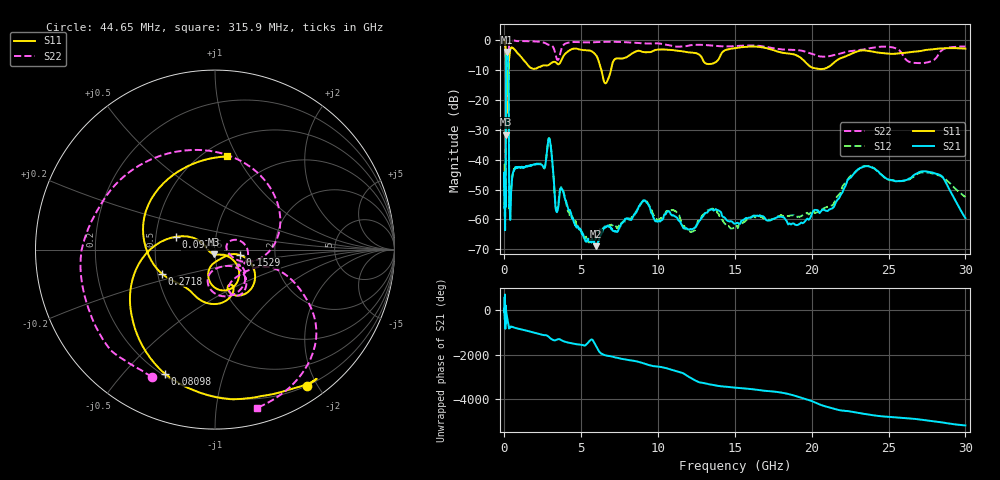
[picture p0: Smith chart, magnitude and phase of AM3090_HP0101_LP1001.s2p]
! Date/Time: Thu, Feb 28, 2019 1:58 PM
! Network Analyzer: Agilent Technologies E8364B Rev: A.07.50.67
! Sweep from 0.010 to 30.000 GHz, 1601 Points, Sweep Type: LOG
! Power Supply: 5.023 V, 0.002 A
# Hz S DB R 50
!freq MagS11 AngS11 MagS21 AngS21 MagS12 AngS12 MagS22 AngS22
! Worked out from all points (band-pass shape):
!   1601 points, 10 MHz to 30 GHz, reference 50 ohm
!   highest |S21| = -3.99 dB at 158.3 MHz (marker M1); lowest = -68.9 dB at 5.959 GHz (marker M2)
!   |S21| within 3 dB of the highest: 107.8 MHz to 249.6 MHz (141.8 MHz wide, 79.3 % of centre)
!   lowest |S11| = -31.6 dB at 105.6 MHz (marker M3), VSWR 1.05, Z = 49.4 - j2.54 ohm
!   |S11| at or under -10 dB: 95.91 MHz to 270.4 MHz (174.5 MHz wide, 95.3 % of centre); 6.308 GHz to 6.931 GHz (622.8 MHz wide, 9.41 % of centre)
!   |S22| runs from -23.8 to -0.1 dB; largest |S21 - S12| = 0.014
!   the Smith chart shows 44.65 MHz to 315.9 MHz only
!   S11 on the Smith chart (normalised r, x): 44.65 MHz: 0.19, -1.86; 80.98 MHz: 0.21, -0.65; 97.46 MHz: 0.64, +0.10; 152.9 MHz: 1.32, -0.08; 271.8 MHz: 0.53, -0.16; 315.9 MHz: 0.63, +0.91
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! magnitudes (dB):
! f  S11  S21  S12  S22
! 10 MHz  -0.2  -44.6  -41.7  -0.8
! 38.04 MHz  -0.5  -60.4  -60.0  -1.6
! 44.65 MHz  -0.8  -58.1  -56.5  -2.0
! 80.98 MHz  -2.6  -50.3  -46.6  -4.8
! 97.46 MHz  -12.9  -15.4  -15.3  -11.8
! 105.6 MHz  -31.6  -7.8  -7.8  -23.5
! 120.9 MHz  -12.7  -5.2  -5.2  -15.7
! 144.7 MHz  -24.2  -4.1  -4.1  -16.4
! 152.9 MHz  -17.0  -4.0  -3.9  -15.4
! 158.3 MHz  -13.6  -4.0  -3.9  -14.0
! 271.8 MHz  -9.8  -15.1  -15.1  -8.6
! 315.9 MHz  -5.6  -55.4  -55.4  -0.8
! 378.2 MHz  -3.2  -60.2  -55.8  -0.3
! 550.5 MHz  -2.7  -44.6  -44.3  -0.2
! 2.084 GHz  -9.5  -41.4  -41.4  -0.5
! 2.928 GHz  -8.1  -33.0  -32.9  -1.6
! 3.385 GHz  -7.6  -57.4  -56.8  -6.0
! 5.959 GHz  -5.0  -68.9  -66.3  -0.7
! 7.926 GHz  -5.8  -59.7  -60.5  -0.7
! 19.12 GHz  -5.4  -61.7  -59.1  -3.4
! 23.59 GHz  -3.5  -42.2  -42.1  -2.9
! 30 GHz  -2.8  -59.5  -52.5  -2.2
